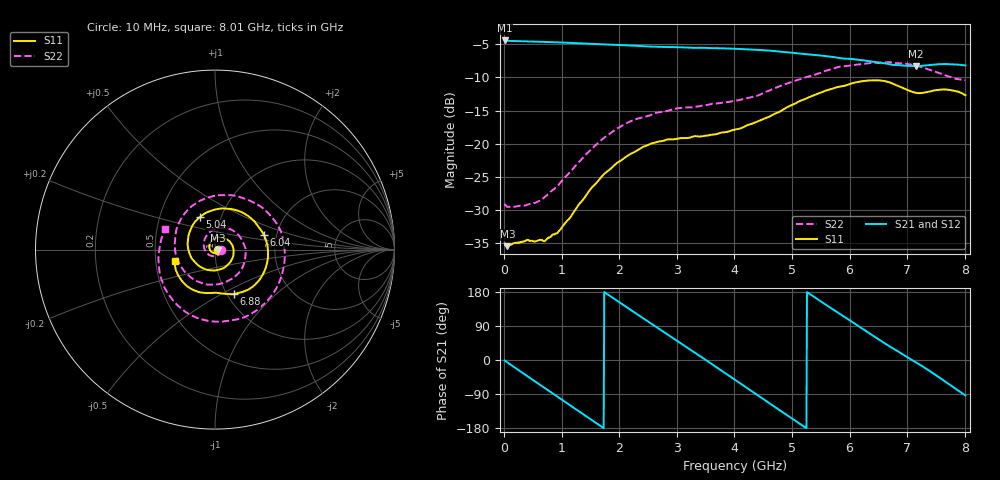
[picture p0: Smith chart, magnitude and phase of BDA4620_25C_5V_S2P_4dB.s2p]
!Agilent Technologies,E5071B,MY42404982,A.09.10
!Date: Wed May 06 08:58:56 2026
!Data & Calibration Information:
!Freq	S11:SOLT2(ON)	S21:SOLT2(ON)	S12:SOLT2(ON)	S22:SOLT2(ON)
# Hz S RI R 50
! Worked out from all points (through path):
!   801 points, 10 MHz to 8.01 GHz, reference 50 ohm
!   highest |S21| = -4.45 dB at 10 MHz (marker M1); lowest = -8.3 dB at 7.15 GHz (marker M2)
!   group delay of S21, straight-line fit = 282 ps
!   lowest |S11| = -35.4 dB at 60 MHz (marker M3), VSWR 1.03, Z = 51.7 - j0.176 ohm
!   |S11| at or under -10 dB: start of sweep to end of sweep
!   |S22| runs from -29.5 to -7.7 dB; largest |S21 - S12| = 0.0027
!   S11 on the Smith chart (normalised r, x): 10 MHz: 1.04, -0.00; 5.04 GHz: 0.79, +0.30; 6.04 GHz: 1.72, +0.30; 6.88 GHz: 1.07, -0.57; 8.01 GHz: 0.63, -0.08
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1e7  0.0177 -0.00113  0.5992 -0.0128  0.5995 -0.0131  0.0351 -0.00278
6e7  0.0168 -0.0017  0.5927 -0.0682  0.5937 -0.0694  0.033 -0.00613
3.7e8  0.0146 -0.0115  0.4586 -0.3714  0.4591 -0.3722  0.0187 -0.0289
7.3e8  -0.00164 -0.0189  0.1362 -0.5679  0.1359 -0.5686  -0.0198 -0.0353
1.03e9  -0.0223 -0.00968  -0.1748 -0.5501  -0.1754 -0.5509  -0.0535 -0.00845
1.35e9  -0.032 0.0187  -0.4415 -0.3608  -0.4417 -0.3615  -0.0609 0.0467
1.64e9  -0.0181 0.0498  -0.5548 -0.0924  -0.5556 -0.0928  -0.0287 0.0978
1.94e9  0.0179 0.0681  -0.5174 0.2012  -0.518 0.2014  0.0396 0.1219
2.33e9  0.0738 0.0514  -0.263 0.4774  -0.2638 0.4777  0.1338 0.0779
2.68e9  0.1039 -0.00109  0.0599 0.534  0.0603 0.5344  0.1714 -0.0151
3e9  0.091 -0.0596  0.3343 0.4158  0.3347 0.4157  0.1466 -0.1116
3.39e9  0.035 -0.1078  0.5173 0.1058  0.5178 0.1048  0.0372 -0.1879
4.01e9  -0.0911 -0.0894  0.3176 -0.4102  0.3171 -0.411  -0.1828 -0.105
4.5e9  -0.1519 0.0216  -0.1135 -0.4934  -0.1139 -0.4941  -0.2163 0.1064
5.04e9  -0.0855 0.1801  -0.4496 -0.1763  -0.4499 -0.1754  -0.0184 0.2957
5.35e9  0.0258 0.2282  -0.4598 0.0812  -0.46 0.0819  0.1532 0.2877
6.04e9  0.2738 0.0793  -0.0809 0.4268  -0.0802 0.4272  0.3887 -0.0292
6.68e9  0.1903 -0.2201  0.3157 0.2407  0.3167 0.2404  0.18 -0.3689
6.88e9  0.1034 -0.2476  0.3689 0.126  0.3703 0.1252  0.049 -0.4003
7.15e9  0.0151 -0.2412  0.3812 -0.0412  0.382 -0.0421  -0.1355 -0.3646
7.57e9  -0.1226 -0.2239  0.2686 -0.2931  0.2692 -0.2941  -0.3024 -0.1518
8.01e9  -0.2233 -0.0621  -0.0235 -0.3875  -0.0248 -0.3888  -0.2782 0.1142
